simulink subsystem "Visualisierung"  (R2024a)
settings: Solver=VariableStepAuto  StartTime=0.0  StopTime=10.0  RelTol=1e-3
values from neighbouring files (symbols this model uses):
  s = tf('s')    [cds_matlab_intro_part3.m]
undefined symbols (not defined in the file or in its folder): ACD120_80_Rotor, ACD120_80_Stator, deg, Heidenhain_ERN_1080, kg, m, N, Visualisierung, X, Y, Z
libraries: sm_lib x37, fl_lib x7, nesl_utility x7

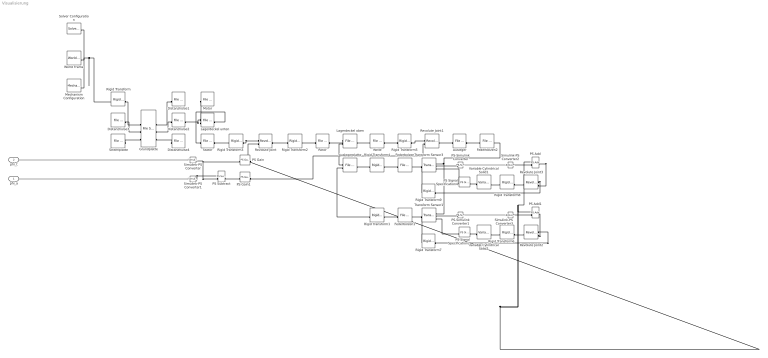
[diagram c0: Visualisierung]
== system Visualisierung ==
  phi_a : Inport
  phi_t : Inport  Port=2
  Ausleger : sm_lib/Body Elements/File Solid  ExtGeomFileName=Visualisierung\Ausleger.par  UnitType=FromFile  ExtGeomFileUnits=m  StepReaderType=HEX  ExportEntireGeometry=off  InertiaType=CalculateFromGeometry  Mass=1  MassUnits=kg  CenterOfMass=[0 0 0]  CenterOfMassUnits=m  MomentsOfInertia=[1 1 1]  MomentsOfInertiaUnits=kg*m^2  ProductsOfInertia=[0 0 0]  ProductsOfInertiaUnits=kg*m^2  BasedOnType=DensityFromFile  Density=7850  DensityUnits=kg/m^3  DoExposeReferenceFrame=off  SerializedFrames=<Frames><Frame><Id>Frame1</Id><Value><Name>F1</Name><Origin><Source>GeometricFeature</Source><FeatureName>circular curve 18</FeatureName></Origin><PrimaryAxis><DefinedDirection>-Z</DefinedDirection><Source>ReferenceFrame</Source><SourceDirection>+Y</SourceDirection><FeatureName></FeatureName></PrimaryAxis><SecondaryAxis><DefinedDirection>+X</DefinedDirection><Source>ReferenceFrame</Source><SourceD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  GraphicType=FromGeometry  MarkerShape=Sphere  MarkerSize=10  GraphicVisPropType=SimpleVisualProperties  GraphicDiffuseColor=[1.0 1.0 0.0]  GraphicSpecularColor=[0.5 0.5 0.5 1.0]  GraphicAmbientColor=[0.15 0.15 0.15 1.0]  GraphicEmissiveColor=[0.0 0.0 0.0 1.0]  GraphicShininess=75  GraphicOpacity=1.0
  Auslegerplatte : sm_lib/Body Elements/File Solid  ExtGeomFileName=Visualisierung\Auslegerplatte.par  UnitType=FromFile  ExtGeomFileUnits=m  StepReaderType=HEX  ExportEntireGeometry=off  InertiaType=CalculateFromGeometry  Mass=1  MassUnits=kg  CenterOfMass=[0 0 0]  CenterOfMassUnits=m  MomentsOfInertia=[1 1 1]  MomentsOfInertiaUnits=kg*m^2  ProductsOfInertia=[0 0 0]  ProductsOfInertiaUnits=kg*m^2  BasedOnType=DensityFromFile  Density=7850  DensityUnits=kg/m^3  DoExposeReferenceFrame=off  SerializedFrames=<Frames><Frame><Id>Frame1</Id><Value><Name>F1</Name><Origin><Source>GeometricFeature</Source><FeatureName>circular curve 22</FeatureName></Origin><PrimaryAxis><DefinedDirection>-Y</DefinedDirection><Source>ReferenceFrame</Source><SourceDirection>+Z</SourceDirection><FeatureName></FeatureName></PrimaryAxis><SecondaryAxis><DefinedDirection>-Z</DefinedDirection><Source>ReferenceFrame</Source><SourceD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  GraphicType=FromGeometry  MarkerShape=Sphere  MarkerSize=10  GraphicVisPropType=SimpleVisualProperties  GraphicDiffuseColor=[0.0 0.4 1.0]  GraphicSpecularColor=[0.5 0.5 0.5 1.0]  GraphicAmbientColor=[0.15 0.15 0.15 1.0]  GraphicEmissiveColor=[0.0 0.0 0.0 1.0]  GraphicShininess=75  GraphicOpacity=1.0
  Distanzhülse1 : sm_lib/Body Elements/File Solid  ExtGeomFileName=Visualisierung\DistanzhuelseGP.par  UnitType=FromFile  ExtGeomFileUnits=m  StepReaderType=HEX  ExportEntireGeometry=off  InertiaType=CalculateFromGeometry  Mass=1  MassUnits=kg  CenterOfMass=[0 0 0]  CenterOfMassUnits=m  MomentsOfInertia=[1 1 1]  MomentsOfInertiaUnits=kg*m^2  ProductsOfInertia=[0 0 0]  ProductsOfInertiaUnits=kg*m^2  BasedOnType=DensityFromFile  Density=7850  DensityUnits=kg/m^3  DoExposeReferenceFrame=on  SerializedFrames=<Frames/>  GraphicType=FromGeometry  MarkerShape=Sphere  MarkerSize=10  GraphicVisPropType=SimpleVisualProperties  GraphicDiffuseColor=[0.0 0.4 1.0]  GraphicSpecularColor=[0.5 0.5 0.5 1.0]  GraphicAmbientColor=[0.15 0.15 0.15 1.0]  GraphicEmissiveColor=[0.0 0.0 0.0 1.0]  GraphicShininess=75  GraphicOpacity=1.0
  Distanzhülse2 : sm_lib/Body Elements/File Solid  ExtGeomFileName=Visualisierung\DistanzhuelseGP.par  UnitType=FromFile  ExtGeomFileUnits=m  StepReaderType=HEX  ExportEntireGeometry=off  InertiaType=CalculateFromGeometry  Mass=1  MassUnits=kg  CenterOfMass=[0 0 0]  CenterOfMassUnits=m  MomentsOfInertia=[1 1 1]  MomentsOfInertiaUnits=kg*m^2  ProductsOfInertia=[0 0 0]  ProductsOfInertiaUnits=kg*m^2  BasedOnType=DensityFromFile  Density=7850  DensityUnits=kg/m^3  DoExposeReferenceFrame=on  SerializedFrames=<Frames><Frame><Id>Frame1</Id><Value><Name>F1</Name><Origin><Source>GeometricFeature</Source><FeatureName>planar surface 1</FeatureName></Origin><PrimaryAxis><DefinedDirection>+Z</DefinedDirection><Source>ReferenceFrame</Source><SourceDirection>+Z</SourceDirection><FeatureName></FeatureName></PrimaryAxis><SecondaryAxis><DefinedDirection>+X</DefinedDirection><Source>ReferenceFrame</Source><SourceDi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  GraphicType=FromGeometry  MarkerShape=Sphere  MarkerSize=10  GraphicVisPropType=SimpleVisualProperties  GraphicDiffuseColor=[0.0 0.4 1.0]  GraphicSpecularColor=[0.5 0.5 0.5 1.0]  GraphicAmbientColor=[0.15 0.15 0.15 1.0]  GraphicEmissiveColor=[0.0 0.0 0.0 1.0]  GraphicShininess=75  GraphicOpacity=1.0
  Distanzhülse3 : sm_lib/Body Elements/File Solid  ExtGeomFileName=Visualisierung\DistanzhuelseGP.par  UnitType=FromFile  ExtGeomFileUnits=m  StepReaderType=HEX  ExportEntireGeometry=off  InertiaType=CalculateFromGeometry  Mass=1  MassUnits=kg  CenterOfMass=[0 0 0]  CenterOfMassUnits=m  MomentsOfInertia=[1 1 1]  MomentsOfInertiaUnits=kg*m^2  ProductsOfInertia=[0 0 0]  ProductsOfInertiaUnits=kg*m^2  BasedOnType=DensityFromFile  Density=7850  DensityUnits=kg/m^3  DoExposeReferenceFrame=on  SerializedFrames=<Frames/>  GraphicType=FromGeometry  MarkerShape=Sphere  MarkerSize=10  GraphicVisPropType=SimpleVisualProperties  GraphicDiffuseColor=[0.0 0.4 1.0]  GraphicSpecularColor=[0.5 0.5 0.5 1.0]  GraphicAmbientColor=[0.15 0.15 0.15 1.0]  GraphicEmissiveColor=[0.0 0.0 0.0 1.0]  GraphicShininess=75  GraphicOpacity=1.0
  Distanzhülse4 : sm_lib/Body Elements/File Solid  ExtGeomFileName=Visualisierung\DistanzhuelseGP.par  UnitType=FromFile  ExtGeomFileUnits=m  StepReaderType=HEX  ExportEntireGeometry=off  InertiaType=CalculateFromGeometry  Mass=1  MassUnits=kg  CenterOfMass=[0 0 0]  CenterOfMassUnits=m  MomentsOfInertia=[1 1 1]  MomentsOfInertiaUnits=kg*m^2  ProductsOfInertia=[0 0 0]  ProductsOfInertiaUnits=kg*m^2  BasedOnType=DensityFromFile  Density=7850  DensityUnits=kg/m^3  DoExposeReferenceFrame=on  SerializedFrames=<Frames/>  GraphicType=FromGeometry  MarkerShape=Sphere  MarkerSize=10  GraphicVisPropType=SimpleVisualProperties  GraphicDiffuseColor=[0.0 0.4 1.0]  GraphicSpecularColor=[0.5 0.5 0.5 1.0]  GraphicAmbientColor=[0.15 0.15 0.15 1.0]  GraphicEmissiveColor=[0.0 0.0 0.0 1.0]  GraphicShininess=75  GraphicOpacity=1.0
  Federbolzen : sm_lib/Body Elements/File Solid  ExtGeomFileName=Visualisierung\Federbolzen.par  UnitType=FromFile  ExtGeomFileUnits=m  StepReaderType=HEX  ExportEntireGeometry=off  InertiaType=CalculateFromGeometry  Mass=1  MassUnits=kg  CenterOfMass=[0 0 0]  CenterOfMassUnits=m  MomentsOfInertia=[1 1 1]  MomentsOfInertiaUnits=kg*m^2  ProductsOfInertia=[0 0 0]  ProductsOfInertiaUnits=kg*m^2  BasedOnType=Density  Density=1  DensityUnits=kg/m^3  DoExposeReferenceFrame=off  SerializedFrames=<Frames><Frame><Id>Frame1</Id><Value><Name>F1</Name><Origin><Source>GeometricFeature</Source><FeatureName>planar surface 3</FeatureName></Origin><PrimaryAxis><DefinedDirection>+Y</DefinedDirection><Source>ReferenceFrame</Source><SourceDirection>+Z</SourceDirection><FeatureName></FeatureName></PrimaryAxis><SecondaryAxis><DefinedDirection>+X</DefinedDirection><Source>ReferenceFrame</Source><SourceDi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  GraphicType=FromGeometry  MarkerShape=Sphere  MarkerSize=10  GraphicVisPropType=SimpleVisualProperties  GraphicDiffuseColor=[0.5 0.5 0.5]  GraphicSpecularColor=[0.5 0.5 0.5 1.0]  GraphicAmbientColor=[0.15 0.15 0.15 1.0]  GraphicEmissiveColor=[0.0 0.0 0.0 1.0]  GraphicShininess=75  GraphicOpacity=1.0
  Federbolzen1 : sm_lib/Body Elements/File Solid  ExtGeomFileName=Visualisierung\Federbolzen.par  UnitType=FromFile  ExtGeomFileUnits=m  StepReaderType=HEX  ExportEntireGeometry=off  InertiaType=CalculateFromGeometry  Mass=1  MassUnits=kg  CenterOfMass=[0 0 0]  CenterOfMassUnits=m  MomentsOfInertia=[1 1 1]  MomentsOfInertiaUnits=kg*m^2  ProductsOfInertia=[0 0 0]  ProductsOfInertiaUnits=kg*m^2  BasedOnType=Density  Density=1  DensityUnits=kg/m^3  DoExposeReferenceFrame=off  SerializedFrames=<Frames><Frame><Id>Frame1</Id><Value><Name>F1</Name><Origin><Source>GeometricFeature</Source><FeatureName>planar surface 3</FeatureName></Origin><PrimaryAxis><DefinedDirection>+Y</DefinedDirection><Source>ReferenceFrame</Source><SourceDirection>+Z</SourceDirection><FeatureName></FeatureName></PrimaryAxis><SecondaryAxis><DefinedDirection>+X</DefinedDirection><Source>ReferenceFrame</Source><SourceDi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  GraphicType=FromGeometry  MarkerShape=Sphere  MarkerSize=10  GraphicVisPropType=SimpleVisualProperties  GraphicDiffuseColor=[0.5 0.5 0.5]  GraphicSpecularColor=[0.5 0.5 0.5 1.0]  GraphicAmbientColor=[0.15 0.15 0.15 1.0]  GraphicEmissiveColor=[0.0 0.0 0.0 1.0]  GraphicShininess=75  GraphicOpacity=1.0
  Federbolzen2 : sm_lib/Body Elements/File Solid  ExtGeomFileName=Visualisierung\Federbolzen.par  UnitType=FromFile  ExtGeomFileUnits=m  StepReaderType=HEX  ExportEntireGeometry=off  InertiaType=CalculateFromGeometry  Mass=1  MassUnits=kg  CenterOfMass=[0 0 0]  CenterOfMassUnits=m  MomentsOfInertia=[1 1 1]  MomentsOfInertiaUnits=kg*m^2  ProductsOfInertia=[0 0 0]  ProductsOfInertiaUnits=kg*m^2  BasedOnType=Density  Density=1  DensityUnits=kg/m^3  DoExposeReferenceFrame=off  SerializedFrames=<Frames><Frame><Id>Frame1</Id><Value><Name>F1</Name><Origin><Source>GeometricFeature</Source><FeatureName>planar surface 3</FeatureName></Origin><PrimaryAxis><DefinedDirection>+Y</DefinedDirection><Source>ReferenceFrame</Source><SourceDirection>+Z</SourceDirection><FeatureName></FeatureName></PrimaryAxis><SecondaryAxis><DefinedDirection>+X</DefinedDirection><Source>ReferenceFrame</Source><SourceDi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  GraphicType=FromGeometry  MarkerShape=Sphere  MarkerSize=10  GraphicVisPropType=SimpleVisualProperties  GraphicDiffuseColor=[0.5 0.5 0.5]  GraphicSpecularColor=[0.5 0.5 0.5 1.0]  GraphicAmbientColor=[0.15 0.15 0.15 1.0]  GraphicEmissiveColor=[0.0 0.0 0.0 1.0]  GraphicShininess=75  GraphicOpacity=1.0
  Grundplatte : sm_lib/Body Elements/File Solid  ExtGeomFileName=Visualisierung\Grundplatte.par  UnitType=FromFile  ExtGeomFileUnits=m  StepReaderType=HEX  ExportEntireGeometry=off  InertiaType=CalculateFromGeometry  Mass=1  MassUnits=kg  CenterOfMass=[0 0 0]  CenterOfMassUnits=m  MomentsOfInertia=[1 1 1]  MomentsOfInertiaUnits=kg*m^2  ProductsOfInertia=[0 0 0]  ProductsOfInertiaUnits=kg*m^2  BasedOnType=DensityFromFile  Density=1  DensityUnits=kg/m^3  DoExposeReferenceFrame=on  SerializedFrames=<Frames><Frame><Id>Frame1</Id><Value><Name>F1</Name><Origin><Source>GeometricFeature</Source><FeatureName>circular curve 15</FeatureName></Origin><PrimaryAxis><DefinedDirection>-Y</DefinedDirection><Source>ReferenceFrame</Source><SourceDirection>+Z</SourceDirection><FeatureName></FeatureName></PrimaryAxis><SecondaryAxis><DefinedDirection>-X</DefinedDirection><Source>ReferenceFrame</Source><SourceD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  GraphicType=FromGeometry  MarkerShape=Sphere  MarkerSize=10  GraphicVisPropType=SimpleVisualProperties  GraphicDiffuseColor=[0.0 0.4 1.0]  GraphicSpecularColor=[0.5 0.5 0.5 1.0]  GraphicAmbientColor=[0.15 0.15 0.15 1.0]  GraphicEmissiveColor=[0.0 0.0 0.0 1.0]  GraphicShininess=75  GraphicOpacity=1.0
  Lagerdeckel oben : sm_lib/Body Elements/File Solid  ExtGeomFileName=Visualisierung\Lagerdeckel_oben.par  UnitType=FromFile  ExtGeomFileUnits=m  StepReaderType=HEX  ExportEntireGeometry=off  InertiaType=CalculateFromGeometry  Mass=1  MassUnits=kg  CenterOfMass=[0 0 0]  CenterOfMassUnits=m  MomentsOfInertia=[1 1 1]  MomentsOfInertiaUnits=kg*m^2  ProductsOfInertia=[0 0 0]  ProductsOfInertiaUnits=kg*m^2  BasedOnType=DensityFromFile  Density=2700  DensityUnits=kg/m^3  DoExposeReferenceFrame=off  SerializedFrames=<Frames><Frame><Id>Frame1</Id><Value><Name>F1</Name><Origin><Source>GeometricFeature</Source><FeatureName>planar surface 2</FeatureName></Origin><PrimaryAxis><DefinedDirection>+Y</DefinedDirection><Source>ReferenceFrame</Source><SourceDirection>+Z</SourceDirection><FeatureName></FeatureName></PrimaryAxis><SecondaryAxis><DefinedDirection>+X</DefinedDirection><Source>ReferenceFrame</Source><SourceDi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  GraphicType=FromGeometry  MarkerShape=Sphere  MarkerSize=10  GraphicVisPropType=SimpleVisualProperties  GraphicDiffuseColor=[1.0 1.0 0.0]  GraphicSpecularColor=[0.5 0.5 0.5 1.0]  GraphicAmbientColor=[0.15 0.15 0.15 1.0]  GraphicEmissiveColor=[0.0 0.0 0.0 1.0]  GraphicShininess=75  GraphicOpacity=1.0
  Lagerdeckel unten : sm_lib/Body Elements/File Solid  ExtGeomFileName=Visualisierung\Lagerdeckel_unten.par  UnitType=FromFile  ExtGeomFileUnits=m  StepReaderType=HEX  ExportEntireGeometry=off  InertiaType=CalculateFromGeometry  Mass=1  MassUnits=kg  CenterOfMass=[0 0 0]  CenterOfMassUnits=m  MomentsOfInertia=[1 1 1]  MomentsOfInertiaUnits=kg*m^2  ProductsOfInertia=[0 0 0]  ProductsOfInertiaUnits=kg*m^2  BasedOnType=DensityFromFile  Density=2700  DensityUnits=kg/m^3  DoExposeReferenceFrame=off  SerializedFrames=<Frames><Frame><Id>Frame1</Id><Value><Name>F1</Name><Origin><Source>GeometricFeature</Source><FeatureName>circular curve 8</FeatureName></Origin><PrimaryAxis><DefinedDirection>-Y</DefinedDirection><Source>ReferenceFrame</Source><SourceDirection>+Z</SourceDirection><FeatureName></FeatureName></PrimaryAxis><SecondaryAxis><DefinedDirection>-X</DefinedDirection><Source>ReferenceFrame</Source><SourceDi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  GraphicType=FromGeometry  MarkerShape=Sphere  MarkerSize=10  GraphicVisPropType=SimpleVisualProperties  GraphicDiffuseColor=[1.0 1.0 0.0]  GraphicSpecularColor=[0.5 0.5 0.5 1.0]  GraphicAmbientColor=[0.15 0.15 0.15 1.0]  GraphicEmissiveColor=[0.0 0.0 0.0 1.0]  GraphicShininess=75  GraphicOpacity=1.0
  Mechanism Configuration : sm_lib/Utilities/Mechanism Configuration  UniformGravity=Constant  GravityVector=[0 0 0]  GravityUnits=m/s^2  LinearizationDelta=0.001
  Motor : sm_lib/Body Elements/File Solid  ExtGeomFileName=Visualisierung\Heidenhain_ERN_1080.par  UnitType=FromFile  ExtGeomFileUnits=m  StepReaderType=HEX  ExportEntireGeometry=off  InertiaType=CalculateFromGeometry  Mass=1  MassUnits=kg  CenterOfMass=[0 0 0]  CenterOfMassUnits=m  MomentsOfInertia=[1 1 1]  MomentsOfInertiaUnits=kg*m^2  ProductsOfInertia=[0 0 0]  ProductsOfInertiaUnits=kg*m^2  BasedOnType=Density  Density=2700  DensityUnits=kg/m^3  DoExposeReferenceFrame=off  SerializedFrames=<Frames><Frame><Id>Frame1</Id><Value><Name>F1</Name><Origin><Source>GeometricFeature</Source><FeatureName>circular curve 17</FeatureName></Origin><PrimaryAxis><DefinedDirection>+Y</DefinedDirection><Source>ReferenceFrame</Source><SourceDirection>+Z</SourceDirection><FeatureName></FeatureName></PrimaryAxis><SecondaryAxis><DefinedDirection>+X</DefinedDirection><Source>ReferenceFrame</Source><SourceD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  GraphicType=FromGeometry  MarkerShape=Sphere  MarkerSize=10  GraphicVisPropType=SimpleVisualProperties  GraphicDiffuseColor=[1 1 1]  GraphicSpecularColor=[0.5 0.5 0.5 1.0]  GraphicAmbientColor=[0.15 0.15 0.15 1.0]  GraphicEmissiveColor=[0.0 0.0 0.0 1.0]  GraphicShininess=75  GraphicOpacity=1.0
  PS Add : fl_lib/Physical Signals/Functions/PS Add
  PS Add1 : fl_lib/Physical Signals/Functions/PS Add
  PS Gain : fl_lib/Physical Signals/Functions/PS Gain  gain=-1
  PS Gain1 : fl_lib/Physical Signals/Functions/PS Gain  gain=-1
  PS Signal Specification2 : fl_lib/Physical Signals/Utilities/PS Signal Specification  signalType=zeros(1, 1) m
  PS Signal Specification4 : fl_lib/Physical Signals/Utilities/PS Signal Specification  signalType=zeros(1, 1) m
  PS Subtract : fl_lib/Physical Signals/Functions/PS Subtract
  PS-Simulink Converter : nesl_utility/PS-Simulink Converter  PhysicalDomain=network_engine_domain  SubClassName=ps_output  LeftPortType=input  RightPortType=output  PseudoPeriodic=off  Frequencies=[]  Unit=inherit  AffineConversion=off
  PS-Simulink Converter1 : nesl_utility/PS-Simulink Converter  PhysicalDomain=network_engine_domain  SubClassName=ps_output  LeftPortType=input  RightPortType=output  PseudoPeriodic=off  Frequencies=[]  Unit=inherit  AffineConversion=off
  Revolute Joint{,1..3} (4 alike) : sm_lib/Joints/Revolute Joint  JointMode=Normal  SenseConstraintForce=off  SenseConstraintForceX=off  SenseConstraintForceY=off  SenseConstraintForceZ=off  SenseConstraintTorque=off  SenseConstraintTorqueX=off  SenseConstraintTorqueY=off  SenseConstraintTorqueZ=off  SenseTotalForce=off  SenseTotalForceX=off  SenseTotalForceY=off  SenseTotalForceZ=off  SenseTotalTorque=off  SenseTotalTorqueX=off  SenseTotalTorqueY=off  SenseTotalTorqueZ=off  CompositeWrenchDir=FollowerOnBase  CompositeWrenchFrame=BaseFrame  EquilibriumPosition=0  EquilibriumPositionUnits=deg  SpringStiffness=0  SpringStiffnessUnits=N*m/deg  DampingCoefficient=0  DampingCoefficientUnits=N*m/(deg/s)  TorqueActuationMode=ComputedTorque  MotionActuationMode=InputMotion  SensePosition=off  SenseVelocity=off  SenseAcceleration=off  SenseTorqueForce=off  SenseLowerLimitTorqueForce=off  SenseUpperLimitTorqueForce=off  LowerLimitSpecify=off  LowerLimitBound=-90  LowerLimitBoundUnits=deg  LowerLimitStiffness=1e4  LowerLimitStiffnessUnits=N*m/deg  LowerLimitDamping=10  LowerLimitDampingUnits=N*m/(deg/s)  LowerLimitTransitionRegionWidth=0.1  LowerLimitTransitionRegionWidthUnits=deg  UpperLimitSpecify=off  UpperLimitBound=90  UpperLimitBoundUnits=deg  UpperLimitStiffness=1e4  UpperLimitStiffnessUnits=N*m/deg  UpperLimitDamping=10  UpperLimitDampingUnits=N*m/(deg/s)  UpperLimitTransitionRegionWidth=0.1  UpperLimitTransitionRegionWidthUnits=deg  PositionTargetSpecify=off  PositionTargetPriority=High  PositionTargetValue=0  PositionTargetValueUnits=deg  VelocityTargetSpecify=off  VelocityTargetPriority=High  VelocityTargetValue=0  VelocityTargetValueUnits=deg/s
  Rigid Transform : sm_lib/Frames and Transforms/Rigid Transform  TranslationMethod=None  TranslationStandardOffset=0  TranslationLengthUnit=m  TranslationStandardAxis=+Z  TranslationCartesianOffset=[0 0 0]  TranslationROffset=0  TranslationROffsetUnits=m  TranslationZOffset=0  TranslationZOffsetUnits=m  TranslationThetaOffset=0  TranslationThetaOffsetUnits=deg  RotationMethod=StandardAxis  RotationAngleUnits=deg  RotationStandardAxis=+Y  RotationAngle=180  RotationArbitraryAxis=[0 0 1]  FollAlignAxisA=+Y  BaseAlignAxisA=-Y  FollAlignAxisB=+X  BaseAlignAxisB=-X  RotationSequenceAxes=FollowerAxes  RotationSequence=XYX  RotationSequenceAngles=[0 0 0]  RotationSequenceAnglesUnits=deg  RotationMatrix=[1 0 0; 0 1 0; 0 0 1]
  Rigid Transform1 : sm_lib/Frames and Transforms/Rigid Transform  TranslationMethod=Cartesian  TranslationStandardOffset=0  TranslationLengthUnit=m  TranslationStandardAxis=+Z  TranslationCartesianOffset=[0 14e-3 0]  TranslationROffset=0  TranslationROffsetUnits=m  TranslationZOffset=0  TranslationZOffsetUnits=m  TranslationThetaOffset=0  TranslationThetaOffsetUnits=deg  RotationMethod=None  RotationAngleUnits=deg  RotationStandardAxis=-X  RotationAngle=90  RotationArbitraryAxis=[0 0 1]  FollAlignAxisA=+Z  BaseAlignAxisA=+Y  FollAlignAxisB=+Y  BaseAlignAxisB=+Z  RotationSequenceAxes=FollowerAxes  RotationSequence=XYX  RotationSequenceAngles=[0 0 0]  RotationSequenceAnglesUnits=deg  RotationMatrix=[1 0 0; 0 1 0; 0 0 1]
  Rigid Transform2 : sm_lib/Frames and Transforms/Rigid Transform  TranslationMethod=None  TranslationStandardOffset=0  TranslationLengthUnit=m  TranslationStandardAxis=+Z  TranslationCartesianOffset=[0 0 0]  TranslationROffset=0  TranslationROffsetUnits=m  TranslationZOffset=0  TranslationZOffsetUnits=m  TranslationThetaOffset=0  TranslationThetaOffsetUnits=deg  RotationMethod=StandardAxis  RotationAngleUnits=deg  RotationStandardAxis=-X  RotationAngle=90  RotationArbitraryAxis=[0 0 1]  FollAlignAxisA=+Z  BaseAlignAxisA=+Y  FollAlignAxisB=+Y  BaseAlignAxisB=+Z  RotationSequenceAxes=FollowerAxes  RotationSequence=XYX  RotationSequenceAngles=[0 0 0]  RotationSequenceAnglesUnits=deg  RotationMatrix=[1 0 0; 0 1 0; 0 0 1]
  Rigid Transform3 : sm_lib/Frames and Transforms/Rigid Transform  TranslationMethod=None  TranslationStandardOffset=0  TranslationLengthUnit=m  TranslationStandardAxis=+Z  TranslationCartesianOffset=[0 0 0]  TranslationROffset=0  TranslationROffsetUnits=m  TranslationZOffset=0  TranslationZOffsetUnits=m  TranslationThetaOffset=0  TranslationThetaOffsetUnits=deg  RotationMethod=StandardAxis  RotationAngleUnits=deg  RotationStandardAxis=+X  RotationAngle=90  RotationArbitraryAxis=[0 0 1]  FollAlignAxisA=+Z  BaseAlignAxisA=+Y  FollAlignAxisB=+Y  BaseAlignAxisB=+Z  RotationSequenceAxes=FollowerAxes  RotationSequence=XYX  RotationSequenceAngles=[0 0 0]  RotationSequenceAnglesUnits=deg  RotationMatrix=[1 0 0; 0 1 0; 0 0 1]
  Rigid Transform4 : sm_lib/Frames and Transforms/Rigid Transform  TranslationMethod=Cartesian  TranslationStandardOffset=0  TranslationLengthUnit=m  TranslationStandardAxis=+Z  TranslationCartesianOffset=[0 14e-3 0]  TranslationROffset=0  TranslationROffsetUnits=m  TranslationZOffset=0  TranslationZOffsetUnits=m  TranslationThetaOffset=0  TranslationThetaOffsetUnits=deg  RotationMethod=None  RotationAngleUnits=deg  RotationStandardAxis=-X  RotationAngle=90  RotationArbitraryAxis=[0 0 1]  FollAlignAxisA=+Z  BaseAlignAxisA=+Y  FollAlignAxisB=+Y  BaseAlignAxisB=+Z  RotationSequenceAxes=FollowerAxes  RotationSequence=XYX  RotationSequenceAngles=[0 0 0]  RotationSequenceAnglesUnits=deg  RotationMatrix=[1 0 0; 0 1 0; 0 0 1]
  Rigid Transform5 : sm_lib/Frames and Transforms/Rigid Transform  TranslationMethod=None  TranslationStandardOffset=0  TranslationLengthUnit=m  TranslationStandardAxis=+Z  TranslationCartesianOffset=[0 0 0]  TranslationROffset=0  TranslationROffsetUnits=m  TranslationZOffset=0  TranslationZOffsetUnits=m  TranslationThetaOffset=0  TranslationThetaOffsetUnits=deg  RotationMethod=StandardAxis  RotationAngleUnits=deg  RotationStandardAxis=+X  RotationAngle=90  RotationArbitraryAxis=[0 0 1]  FollAlignAxisA=+Z  BaseAlignAxisA=+Y  FollAlignAxisB=+Y  BaseAlignAxisB=+Z  RotationSequenceAxes=FollowerAxes  RotationSequence=XYX  RotationSequenceAngles=[0 0 0]  RotationSequenceAnglesUnits=deg  RotationMatrix=[1 0 0; 0 1 0; 0 0 1]
  Rigid Transform6 : sm_lib/Frames and Transforms/Rigid Transform  TranslationMethod=None  TranslationStandardOffset=0  TranslationLengthUnit=m  TranslationStandardAxis=+Z  TranslationCartesianOffset=[0 0 0]  TranslationROffset=0  TranslationROffsetUnits=m  TranslationZOffset=0  TranslationZOffsetUnits=m  TranslationThetaOffset=0  TranslationThetaOffsetUnits=deg  RotationMethod=StandardAxis  RotationAngleUnits=deg  RotationStandardAxis=+Y  RotationAngle=90  RotationArbitraryAxis=[0 0 1]  FollAlignAxisA=+X  BaseAlignAxisA=+Y  FollAlignAxisB=+Z  BaseAlignAxisB=-X  RotationSequenceAxes=FollowerAxes  RotationSequence=XYX  RotationSequenceAngles=[0 0 0]  RotationSequenceAnglesUnits=deg  RotationMatrix=[1 0 0; 0 1 0; 0 0 1]
  Rigid Transform7 : sm_lib/Frames and Transforms/Rigid Transform  TranslationMethod=None  TranslationStandardOffset=0  TranslationLengthUnit=m  TranslationStandardAxis=+Z  TranslationCartesianOffset=[0 0 0]  TranslationROffset=0  TranslationROffsetUnits=m  TranslationZOffset=0  TranslationZOffsetUnits=m  TranslationThetaOffset=0  TranslationThetaOffsetUnits=deg  RotationMethod=StandardAxis  RotationAngleUnits=deg  RotationStandardAxis=+X  RotationAngle=-90  RotationArbitraryAxis=[0 0 1]  FollAlignAxisA=+Z  BaseAlignAxisA=+Y  FollAlignAxisB=+Y  BaseAlignAxisB=+Z  RotationSequenceAxes=FollowerAxes  RotationSequence=XYX  RotationSequenceAngles=[0 0 0]  RotationSequenceAnglesUnits=deg  RotationMatrix=[1 0 0; 0 1 0; 0 0 1]
  Rigid Transform8 : sm_lib/Frames and Transforms/Rigid Transform  TranslationMethod=None  TranslationStandardOffset=0  TranslationLengthUnit=m  TranslationStandardAxis=+Z  TranslationCartesianOffset=[0 0 0]  TranslationROffset=0  TranslationROffsetUnits=m  TranslationZOffset=0  TranslationZOffsetUnits=m  TranslationThetaOffset=0  TranslationThetaOffsetUnits=deg  RotationMethod=StandardAxis  RotationAngleUnits=deg  RotationStandardAxis=+Y  RotationAngle=90  RotationArbitraryAxis=[0 0 1]  FollAlignAxisA=+X  BaseAlignAxisA=+Y  FollAlignAxisB=+Z  BaseAlignAxisB=-X  RotationSequenceAxes=FollowerAxes  RotationSequence=XYX  RotationSequenceAngles=[0 0 0]  RotationSequenceAnglesUnits=deg  RotationMatrix=[1 0 0; 0 1 0; 0 0 1]
  Rigid Transform9 : sm_lib/Frames and Transforms/Rigid Transform  TranslationMethod=None  TranslationStandardOffset=0  TranslationLengthUnit=m  TranslationStandardAxis=+Z  TranslationCartesianOffset=[0 0 0]  TranslationROffset=0  TranslationROffsetUnits=m  TranslationZOffset=0  TranslationZOffsetUnits=m  TranslationThetaOffset=0  TranslationThetaOffsetUnits=deg  RotationMethod=StandardAxis  RotationAngleUnits=deg  RotationStandardAxis=+X  RotationAngle=-90  RotationArbitraryAxis=[0 0 1]  FollAlignAxisA=+Z  BaseAlignAxisA=+Y  FollAlignAxisB=+Y  BaseAlignAxisB=+Z  RotationSequenceAxes=FollowerAxes  RotationSequence=XYX  RotationSequenceAngles=[0 0 0]  RotationSequenceAnglesUnits=deg  RotationMatrix=[1 0 0; 0 1 0; 0 0 1]
  Rotor : sm_lib/Body Elements/File Solid  ExtGeomFileName=Visualisierung\ACD120_80_Rotor.par  UnitType=FromFile  ExtGeomFileUnits=m  StepReaderType=HEX  ExportEntireGeometry=off  InertiaType=CalculateFromGeometry  Mass=1  MassUnits=kg  CenterOfMass=[0 0 0]  CenterOfMassUnits=m  MomentsOfInertia=[1 1 1]  MomentsOfInertiaUnits=kg*m^2  ProductsOfInertia=[0 0 0]  ProductsOfInertiaUnits=kg*m^2  BasedOnType=Density  Density=7850  DensityUnits=kg/m^3  DoExposeReferenceFrame=off  SerializedFrames=<Frames><Frame><Id>Frame1</Id><Value><Name>F1</Name><Origin><Source>GeometricFeature</Source><FeatureName>circular curve 77</FeatureName></Origin><PrimaryAxis><DefinedDirection>+Y</DefinedDirection><Source>ReferenceFrame</Source><SourceDirection>+Z</SourceDirection><FeatureName></FeatureName></PrimaryAxis><SecondaryAxis><DefinedDirection>+X</DefinedDirection><Source>ReferenceFrame</Source><SourceD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  GraphicType=FromGeometry  MarkerShape=Sphere  MarkerSize=10  GraphicVisPropType=SimpleVisualProperties  GraphicDiffuseColor=[0.4 0.4 0.4]  GraphicSpecularColor=[0.5 0.5 0.5 1.0]  GraphicAmbientColor=[0.15 0.15 0.15 1.0]  GraphicEmissiveColor=[0.0 0.0 0.0 1.0]  GraphicShininess=75  GraphicOpacity=1.0
  Seitenplatte : sm_lib/Body Elements/File Solid  ExtGeomFileName=Visualisierung\Seitenplatte.par  UnitType=FromFile  ExtGeomFileUnits=m  StepReaderType=HEX  ExportEntireGeometry=off  InertiaType=CalculateFromGeometry  Mass=1  MassUnits=kg  CenterOfMass=[0 0 0]  CenterOfMassUnits=m  MomentsOfInertia=[1 1 1]  MomentsOfInertiaUnits=kg*m^2  ProductsOfInertia=[0 0 0]  ProductsOfInertiaUnits=kg*m^2  BasedOnType=DensityFromFile  Density=1  DensityUnits=kg/m^3  DoExposeReferenceFrame=off  SerializedFrames=<Frames><Frame><Id>Frame1</Id><Value><Name>F1</Name><Origin><Source>GeometricFeature</Source><FeatureName>segment 13</FeatureName></Origin><PrimaryAxis><DefinedDirection>-Y</DefinedDirection><Source>ReferenceFrame</Source><SourceDirection>+X</SourceDirection><FeatureName></FeatureName></PrimaryAxis><SecondaryAxis><DefinedDirection>+X</DefinedDirection><Source>ReferenceFrame</Source><SourceDirectio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  GraphicType=FromGeometry  MarkerShape=Sphere  MarkerSize=10  GraphicVisPropType=SimpleVisualProperties  GraphicDiffuseColor=[0.0 0.4 1.0]  GraphicSpecularColor=[0.5 0.5 0.5 1.0]  GraphicAmbientColor=[0.15 0.15 0.15 1.0]  GraphicEmissiveColor=[0.0 0.0 0.0 1.0]  GraphicShininess=75  GraphicOpacity=1.0
  Simulink-PS Converter{,1..3} (4 alike) : nesl_utility/Simulink-PS Converter  PhysicalDomain=network_engine_domain  SubClassName=ps_input  LeftPortType=input  RightPortType=output  PseudoPeriodic=off  Frequencies=[]  NoiseDistribution=none  NoiseParameters=[]  Unit=1  AffineConversion=off  FilteringAndDerivatives=filter  SimscapeFilterOrder=2  InputFilterTimeConstant=0.001  UdotUserProvided=0
  Solver Configuration : nesl_utility/Solver Configuration  PhysicalDomain=network_engine_domain  SubClassName=solver  LeftPortType=input  RightPortType=generic  Tones=[]  Harmonics=[]  SimulateNoise=off  Profile=off  UseLocalSampling=off  EnableSwitchedLinearOptims=on  FrequencyDomain=off  UseCCode=off  RelTol=0.001  AbsTol=1e-06  MinStep=1e-09  ToWorkspace=off  RevertToSquareIcSolve=off  NumHomotopyIterations=100  PhasorMode=off  PhasorModeNumHarmonics=1  DoDC=off  ResidualTolerance=1e-09  UseLocalSolver=off  LocalSolverChoice=NE_BACKWARD_EULER_ADVANCER  LocalSolverSampleTime=0.001  DoFixedCost=off  MaxNonlinIter=3  MaxModeIter=2  LinearAlgebra=Sparse  EquationFormulation=NE_TIME_EF  DelaysMemoryBudget=1024  AutomaticFiltering=on  FilteringTimeConstant=0.001  PartitionStorageMethod=AS_NEEDED  PartitionMemoryBudget=1024  PartitionMethod=FAST
  Stator : sm_lib/Body Elements/File Solid  ExtGeomFileName=Visualisierung\ACD120_80_Stator.par  UnitType=FromFile  ExtGeomFileUnits=m  StepReaderType=HEX  ExportEntireGeometry=off  InertiaType=CalculateFromGeometry  Mass=1  MassUnits=kg  CenterOfMass=[0 0 0]  CenterOfMassUnits=m  MomentsOfInertia=[1 1 1]  MomentsOfInertiaUnits=kg*m^2  ProductsOfInertia=[0 0 0]  ProductsOfInertiaUnits=kg*m^2  BasedOnType=Density  Density=7850  DensityUnits=kg/m^3  DoExposeReferenceFrame=off  SerializedFrames=<Frames><Frame><Id>Frame1</Id><Value><Name>F1</Name><Origin><Source>GeometricFeature</Source><FeatureName>planar surface 22</FeatureName></Origin><PrimaryAxis><DefinedDirection>+Y</DefinedDirection><Source>ReferenceFrame</Source><SourceDirection>+Z</SourceDirection><FeatureName></FeatureName></PrimaryAxis><SecondaryAxis><DefinedDirection>-Z</DefinedDirection><Source>ReferenceFrame</Source><SourceD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  GraphicType=FromGeometry  MarkerShape=Sphere  MarkerSize=10  GraphicVisPropType=SimpleVisualProperties  GraphicDiffuseColor=[0.4 0.4 0.4]  GraphicSpecularColor=[0.5 0.5 0.5 1.0]  GraphicAmbientColor=[0.15 0.15 0.15 1.0]  GraphicEmissiveColor=[0.0 0.0 0.0 1.0]  GraphicShininess=75  GraphicOpacity=1.0
  Transform Sensor1 : sm_lib/Frames and Transforms/Transform Sensor  MeasurementFrame=World  SenseAngle=off  SenseAxis=off  SenseAngle1=off  SenseAngle2=off  SenseAngle3=off  SenseQ=off  SenseR=off  SenseOmegaX=off  SenseOmegaY=off  SenseOmegaZ=off  SenseOmega1=off  SenseOmega2=off  SenseOmega3=off  SenseQDot=off  SenseRDot=off  SenseAlphaX=off  SenseAlphaY=off  SenseAlphaZ=off  SenseAlpha1=off  SenseAlpha2=off  SenseAlpha3=off  SenseQDDot=off  SenseRDDot=off  SenseX=off  SenseY=off  SenseZ=off  SenseRad=off  SenseAzim=on  SenseDist=on  SenseInc=off  SenseXDot=off  SenseYDot=off  SenseZDot=off  SenseRadDot=off  SenseAzimDot=off  SenseDistDot=off  SenseIncDot=off  SenseXDDot=off  SenseYDDot=off  SenseZDDot=off  SenseRadDDot=off  SenseAzimDDot=off  SenseDistDDot=off  SenseIncDDot=off
  Transform Sensor3 : sm_lib/Frames and Transforms/Transform Sensor  MeasurementFrame=World  SenseAngle=off  SenseAxis=off  SenseAngle1=off  SenseAngle2=off  SenseAngle3=off  SenseQ=off  SenseR=off  SenseOmegaX=off  SenseOmegaY=off  SenseOmegaZ=off  SenseOmega1=off  SenseOmega2=off  SenseOmega3=off  SenseQDot=off  SenseRDot=off  SenseAlphaX=off  SenseAlphaY=off  SenseAlphaZ=off  SenseAlpha1=off  SenseAlpha2=off  SenseAlpha3=off  SenseQDDot=off  SenseRDDot=off  SenseX=off  SenseY=off  SenseZ=off  SenseRad=off  SenseAzim=on  SenseDist=on  SenseInc=off  SenseXDot=off  SenseYDot=off  SenseZDot=off  SenseRadDot=off  SenseAzimDot=off  SenseDistDot=off  SenseIncDot=off  SenseXDDot=off  SenseYDDot=off  SenseZDDot=off  SenseRadDDot=off  SenseAzimDDot=off  SenseDistDDot=off  SenseIncDDot=off
  Variable Cylindrical Solid1 : sm_lib/Body Elements/Variable Mass/Variable Cylindrical Solid  LengthType=ProvidedByInput  Length=1  LengthUnits=m  RadiusType=Constant  Radius=2.5e-3  RadiusUnits=m  MassType=CalculateFromGeometry  InitialMassType=Specified  InitialMass=1  InitialMassUnits=kg  Density=1000  DensityUnits=kg/m^3  SenseRadius=off  SenseLength=off  SenseMass=off  SenseCenterOfMass=off  SenseInertiaMatrix=off  GraphicType=FromGeometry  MarkerShape=Sphere  MarkerSize=10  GraphicVisPropType=SimpleVisualProperties  GraphicDiffuseColor=[1.0 1.0 1.0]  GraphicSpecularColor=[0.5 0.5 0.5 1.0]  GraphicAmbientColor=[0.15 0.15 0.15 1.0]  GraphicEmissiveColor=[0.0 0.0 0.0 1.0]  GraphicShininess=75  GraphicOpacity=1.0
  Variable Cylindrical Solid2 : sm_lib/Body Elements/Variable Mass/Variable Cylindrical Solid  LengthType=ProvidedByInput  Length=1  LengthUnits=m  RadiusType=Constant  Radius=2.5e-3  RadiusUnits=m  MassType=CalculateFromGeometry  InitialMassType=Specified  InitialMass=1  InitialMassUnits=kg  Density=1000  DensityUnits=kg/m^3  SenseRadius=off  SenseLength=off  SenseMass=off  SenseCenterOfMass=off  SenseInertiaMatrix=off  GraphicType=FromGeometry  MarkerShape=Sphere  MarkerSize=10  GraphicVisPropType=SimpleVisualProperties  GraphicDiffuseColor=[1.0 1.0 1.0]  GraphicSpecularColor=[0.5 0.5 0.5 1.0]  GraphicAmbientColor=[0.15 0.15 0.15 1.0]  GraphicEmissiveColor=[0.0 0.0 0.0 1.0]  GraphicShininess=75  GraphicOpacity=1.0
  Welle : sm_lib/Body Elements/File Solid  ExtGeomFileName=Visualisierung\Welle.par  UnitType=FromFile  ExtGeomFileUnits=m  StepReaderType=HEX  ExportEntireGeometry=off  InertiaType=CalculateFromGeometry  Mass=1  MassUnits=kg  CenterOfMass=[0 0 0]  CenterOfMassUnits=m  MomentsOfInertia=[1 1 1]  MomentsOfInertiaUnits=kg*m^2  ProductsOfInertia=[0 0 0]  ProductsOfInertiaUnits=kg*m^2  BasedOnType=DensityFromFile  Density=1  DensityUnits=kg/m^3  DoExposeReferenceFrame=off  SerializedFrames=<Frames><Frame><Id>Frame1</Id><Value><Name>F1</Name><Origin><Source>GeometricFeature</Source><FeatureName>planar surface 1</FeatureName></Origin><PrimaryAxis><DefinedDirection>+Y</DefinedDirection><Source>ReferenceFrame</Source><SourceDirection>+Z</SourceDirection><FeatureName></FeatureName></PrimaryAxis><SecondaryAxis><DefinedDirection>-X</DefinedDirection><Source>ReferenceFrame</Source><SourceDi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  GraphicType=FromGeometry  MarkerShape=Sphere  MarkerSize=10  GraphicVisPropType=SimpleVisualProperties  GraphicDiffuseColor=[0.5 0.5 0.5]  GraphicSpecularColor=[0.5 0.5 0.5 1.0]  GraphicAmbientColor=[0.15 0.15 0.15 1.0]  GraphicEmissiveColor=[0.0 0.0 0.0 1.0]  GraphicShininess=75  GraphicOpacity=1.0
  World Frame : sm_lib/Frames and Transforms/World Frame
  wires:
  phi_t/1 -> Simulink-PS Converter/1
  phi_a/1 -> Simulink-PS Converter1/1
  PS-Simulink Converter/1 -> Simulink-PS Converter2/1
  PS-Simulink Converter1/1 -> Simulink-PS Converter3/1
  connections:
  World Frame/RConn1 -- Mechanism Configuration/RConn1 -- Rigid Transform/LConn1 -- Solver Configuration/RConn1
  Auslegerplatte/RConn1 -- Rigid Transform4/LConn1
  Rigid Transform5/LConn1 -- Welle/RConn1
  Welle/LConn1 -- Lagerdeckel oben/RConn1
  Distanzhülse3/RConn1 -- Grundplatte/RConn2
  Auslegerplatte/LConn1 -- Lagerdeckel oben/LConn2
  Rigid Transform5/RConn1 -- Revolute Joint1/LConn1
  Rigid Transform/RConn1 -- Grundplatte/RConn1
  Rigid Transform3/RConn1 -- Revolute Joint/LConn1
  Motor/LConn1 -- Lagerdeckel unten/LConn2
  Distanzhülse1/RConn1 -- Grundplatte/LConn1
  Rigid Transform1/RConn1 -- Federbolzen1/LConn1
  Lagerdeckel unten/LConn1 -- Distanzhülse2/LConn1
  Federbolzen/LConn1 -- Rigid Transform4/RConn1
  Federbolzen2/LConn1 -- Ausleger/RConn1
  Rotor/LConn1 -- Rigid Transform2/RConn1
  Stator/LConn1 -- Lagerdeckel unten/RConn1
  Revolute Joint/RConn1 -- Rigid Transform2/LConn1
  Lagerdeckel oben/LConn1 -- Rotor/RConn1
  Seitenplatte/LConn1 -- Grundplatte/RConn3
  Rigid Transform1/LConn1 -- Auslegerplatte/LConn2
  Rigid Transform3/LConn1 -- Stator/RConn1
  Distanzhülse2/RConn1 -- Grundplatte/LConn2
  Distanzhülse4/RConn1 -- Grundplatte/LConn3
  Revolute Joint1/RConn1 -- Ausleger/LConn1
  Simulink-PS Converter1/RConn1 -- PS Subtract/LConn1
  Transform Sensor1/LConn1 -- Federbolzen1/RConn1 -- Rigid Transform7/LConn1
  Transform Sensor3/LConn1 -- Federbolzen/RConn1 -- Rigid Transform9/LConn1
  Transform Sensor1/RConn1 -- Federbolzen2/RConn1 -- Transform Sensor3/RConn1
  Simulink-PS Converter2/RConn1 -- PS Add/LConn2
  Simulink-PS Converter3/RConn1 -- PS Add1/LConn2
  Revolute Joint2/RConn1 -- Rigid Transform6/LConn1
  Transform Sensor1/RConn2 -- PS-Simulink Converter1/LConn1
  Transform Sensor1/RConn3 -- PS Signal Specification2/LConn1
  Revolute Joint2/LConn1 -- Rigid Transform7/RConn1
  Revolute Joint3/LConn2 -- PS Add/RConn1
  PS Signal Specification4/LConn1 -- Transform Sensor3/RConn3
  PS-Simulink Converter/LConn1 -- Transform Sensor3/RConn2
  Variable Cylindrical Solid1/LConn1 -- PS Signal Specification4/RConn1
  Rigid Transform8/RConn1 -- Variable Cylindrical Solid1/RConn1
  PS Add1/RConn1 -- Revolute Joint2/LConn2
  Variable Cylindrical Solid2/LConn1 -- PS Signal Specification2/RConn1
  Revolute Joint3/RConn1 -- Rigid Transform8/LConn1
  Rigid Transform6/RConn1 -- Variable Cylindrical Solid2/RConn1
  Rigid Transform9/RConn1 -- Revolute Joint3/LConn1
  Revolute Joint1/LConn2 -- PS Gain1/RConn1
  PS Subtract/RConn1 -- PS Gain1/LConn1
  Simulink-PS Converter/RConn1 -- PS Subtract/LConn2 -- PS Gain/LConn1
  PS Gain/RConn1 -- PS Add/LConn1 -- PS Add1/LConn1 -- Revolute Joint/LConn2
